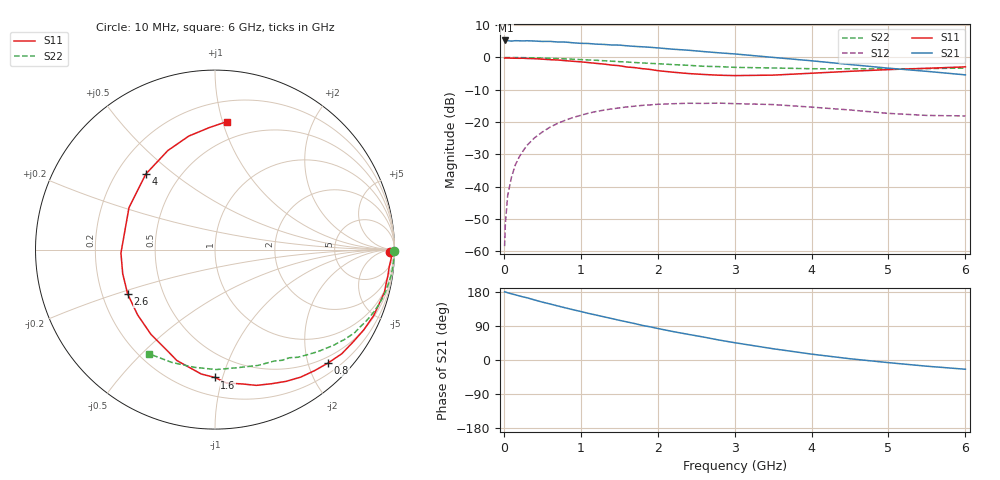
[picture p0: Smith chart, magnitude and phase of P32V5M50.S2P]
! SIEMENS Small Signal Semiconductors
! BFP181
! Si NPN RF Bipolar Junction Transistor in SOT143
! VCE = 2.5 V  IC = 0.5 mA
! Common Emitter S-Parameters:  March  1996
# GHz  S  MA  R  50
!  f  S11  S21  S12  S22
! GHz  MAG  ANG  MAG  ANG  MAG  ANG  MAG  ANG
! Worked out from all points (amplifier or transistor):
!   36 points, 10 MHz to 6 GHz, reference 50 ohm
!   highest |S21| = 5.3 dB at 20 MHz (marker M1)
!   |S21| within 3 dB of that: start of sweep to 2.383 GHz
!   unconditionally stable (mu >= 1): 3.738 GHz to end of sweep
!   at 250 MHz: K = 0.08, MSG = 17.0 dB, |S12| = -28.9 dB
!   at 1.4 GHz: K = 0.43, MSG = 9.9 dB, |S12| = -15.9 dB
!   at 6 GHz: K = 1.46, MAG = 2.3 dB, |S12| = -18.1 dB
!   S11 on the Smith chart (normalised r, x): 10 MHz: 69, -37; 800 MHz: 0.38, -2.36; 1.6 GHz: 0.33, -0.94; 2.6 GHz: 0.31, -0.22; 4 GHz: 0.32, +0.40; 6 GHz: 0.35, +1.03
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0.01  0.9778 -0.7  1.814 179.9  0.0012 87.0  0.9989 -0.3
0.02  0.9785 -1.3  1.835 179.5  0.0027 91.5  0.9988 -0.6
0.05  0.9835 -2.6  1.822 177.4  0.0073 90.9  0.9984 -1.4
0.1  0.9754 -5.7  1.794 174.6  0.0141 85.6  0.9988 -2.8
0.15  0.9742 -8.6  1.82 172.0  0.0218 83.5  0.9963 -4.1
0.2  0.9718 -11.3  1.813 169.2  0.0289 82.3  0.9957 -5.5
0.3  0.9654 -17.2  1.816 164.3  0.0435 78.2  0.992 -8.2
0.4  0.9575 -22.5  1.799 158.4  0.0572 74.2  0.9858 -10.9
0.6  0.9251 -34.0  1.775 147.9  0.0835 65.8  0.9714 -16.2
0.8  0.8925 -45.0  1.733 137.6  0.1068 58.4  0.9516 -21.2
1.1  0.8339 -61.7  1.646 123.0  0.1373 47.6  0.9155 -28.2
1.5  0.746 -85.1  1.556 104.8  0.1658 34.5  0.8619 -36.8
1.6  0.7123 -90.1  1.517 100.5  0.1717 31.8  0.8511 -38.6
1.9  0.6534 -109.0  1.439 87.6  0.1845 23.2  0.8107 -44.2
2.2  0.5919 -127.1  1.343 75.0  0.1924 15.6  0.7764 -49.2
2.6  0.5458 -153.1  1.234 60.4  0.1947 6.9  0.7311 -55.5
3  0.5244 -177.9  1.135 45.7  0.193 -1.6  0.7034 -61.9
3.5  0.5332 154.0  1.003 29.7  0.1868 -9.7  0.688 -69.8
4  0.5707 132.5  0.889 15.5  0.1705 -15.8  0.6699 -79.1
4.5  0.6111 115.5  0.778 3.3  0.154 -20.4  0.6683 -89.4
5.5  0.6804 92.7  0.61 -16.4  0.1268 -16.6  0.6731 -111.1
6  0.7162 84.7  0.538 -24.4  0.1245 -12.5  0.6866 -122.2
